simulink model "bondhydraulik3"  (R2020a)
settings: Solver=ode45  StartTime=0.0  StopTime=2  MaxStep=0.01  RelTol=1e-3  EnableMultiTasking=on
undefined symbols (not defined in the file or in its folder): Display, Int, libbondgraph
libraries: libbondgraph x7

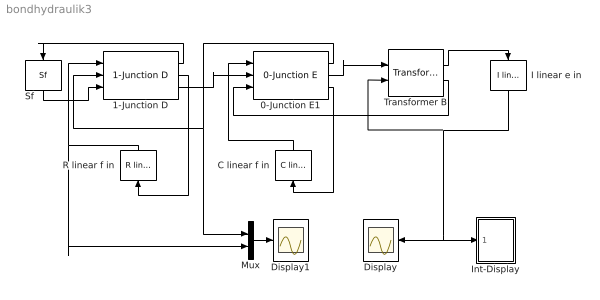
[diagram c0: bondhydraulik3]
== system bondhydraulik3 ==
  0-Junction E1 : libbondgraph/0-Junction E
  1-Junction D : libbondgraph/1-Junction D
  C linear f in : libbondgraph/C linear f in  C=1.74e-12
  Display : Scope
  Display1 : Scope
  I linear e in : libbondgraph/I linear e in  I=500
  Int-Display : Subsystem  AncestorBlock=libbondgraph/Int-Display
  Mux : Mux  Inputs=2
  R linear f in : libbondgraph/R linear f in  R=8e7
  Sf : libbondgraph/Sf  f_ext=0.001
  Transformer B : libbondgraph/Transformer B  m=1000
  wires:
  Transformer B/1 -> I linear e in/1
  I linear e in/1 -> Transformer B/2, Display/1, Int-Display/1(In1)
  Mux/1 -> Display1/1
  0-Junction E1/1 -> Mux/1, 1-Junction D/2
  0-Junction E1/3 -> C linear f in/1
  C linear f in/1 -> 0-Junction E1/1
  0-Junction E1/2 -> Transformer B/1
  Transformer B/2 -> 0-Junction E1/3
  Sf/1 -> 1-Junction D/3
  1-Junction D/1 -> Sf/1
  1-Junction D/2 -> R linear f in/1
  R linear f in/1 -> 1-Junction D/1, Mux/2
  1-Junction D/3 -> 0-Junction E1/2

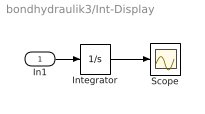
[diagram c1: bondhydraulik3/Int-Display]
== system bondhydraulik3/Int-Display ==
  In1 : Inport
  Integrator : Integrator
  Scope : Scope
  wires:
  Integrator/1 -> Scope/1
  In1/1 -> Integrator/1
